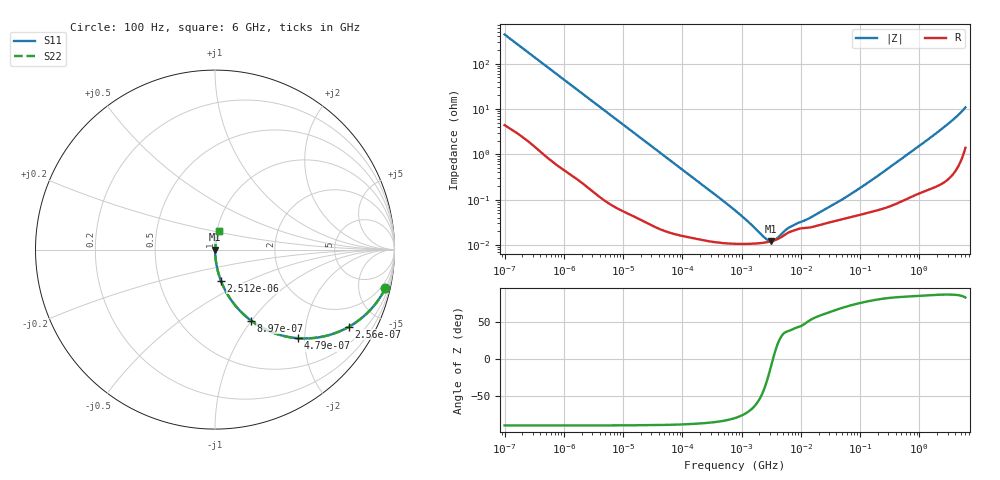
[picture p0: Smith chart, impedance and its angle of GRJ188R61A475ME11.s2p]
!Murata Part Number: GRJ188R61A475ME11
!These Parameters are Measured in Series Mode Connection
!Data Generated on Jun 19, 2026
!  o--ll--o
!Port1  Port2
!  o------o
!Operation Temp=25[degC], DC Bias Voltage=0[V]
!Freq. Start=100[Hz] Stop=6[GHz] 401[Steps]
# Hz S RI R 50
!Freq.(Hz) S11(Real) S11(Imag) S21(Real) S21(Imag) S12(Real) S12(Imag) S22(Real) S22(Imag)
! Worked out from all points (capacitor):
!   401 points, 100 Hz to 6 GHz, reference 50 ohm
!   read as one part in series: C = 3.61 uF near 109 Hz
!   lowest |Z| = 12.3 mohm at 3.104 MHz (marker M1)
!   series resonance near 3.388 MHz, so ESL is about 610 pH
!   S11 on the Smith chart (normalised r, x): 100 Hz: 1.09, -8.81; 256 Hz: 1.04, -3.46; 479 Hz: 1.02, -1.86; 897 Hz: 1.01, -1.00; 2.512 kHz: 1.00, -0.36; 6 GHz: 1.03, +0.22
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100  0.949 -0.215  0.051 0.215  0.051 0.215  0.949 -0.215
164  0.8767 -0.3234  0.1233 0.3234  0.1233 0.3234  0.8767 -0.3234
256  0.7476 -0.4289  0.2524 0.4289  0.2524 0.4289  0.7476 -0.4289
350  0.6157 -0.4812  0.3843 0.4812  0.3843 0.4812  0.6157 -0.4812
479  0.4638 -0.4937  0.5362 0.4937  0.5362 0.4937  0.4638 -0.4937
897  0.2013 -0.396  0.7987 0.396  0.7987 0.396  0.2013 -0.396
1283  0.1111 -0.3091  0.8889 0.3091  0.8889 0.3091  0.1111 -0.3091
2008  0.0497 -0.2121  0.9503 0.2121  0.9503 0.2121  0.0497 -0.2121
2512  0.0328 -0.1729  0.9672 0.1729  0.9672 0.1729  0.0328 -0.1729
7695  0.0041 -0.0585  0.9959 0.0585  0.9959 0.0585  0.0041 -0.0585
40335  0.000358 -0.0113  0.9996 0.0113  0.9996 0.0113  0.000358 -0.0113
774597  0.000107 -0.000573  0.9999 0.000573  0.9999 0.000573  0.000107 -0.000573
1325623  0.000106 -0.000299  0.9999 0.000299  0.9999 0.000299  0.000106 -0.000299
2481164  0.000113 -8.74e-05  0.9999 8.74e-05  0.9999 8.74e-05  0.000113 -8.74e-05
3103719  0.00012 -2.42e-05  0.9999 2.42e-05  0.9999 2.42e-05  0.00012 -2.42e-05
3882480  0.000132 3.71e-05  0.9999 -3.71e-05  0.9999 -3.71e-05  0.000132 3.71e-05
6353432  0.000192 0.000149  0.9998 -0.000149  0.9998 -0.000149  0.000192 0.000149
1.555665e7  0.00025 0.000341  0.9997 -0.000341  0.9997 -0.000341  0.00025 0.000341
6.518806e7  0.000402 0.00119  0.9996 -0.00119  0.9996 -0.00119  0.000402 0.00119
3.124326e8  0.000731 0.00506  0.9993 -0.00506  0.9993 -0.00506  0.000731 0.00506
2.240541e9  0.00327 0.0337  0.9967 -0.0337  0.9967 -0.0337  0.00327 0.0337
6e9  0.0248 0.1038  0.9752 -0.1038  0.9752 -0.1038  0.0248 0.1038
